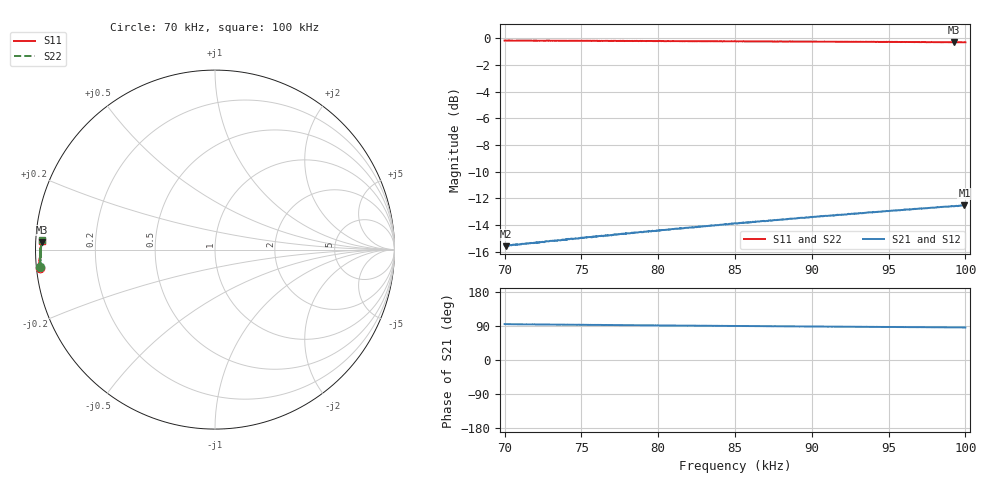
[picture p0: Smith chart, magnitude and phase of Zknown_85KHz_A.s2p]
!Keysight Technologies N9928A: A.12.01
!Date: Monday, January 30, 2023
!Model: N9928A
!Serial: MY58311550
!Caliblation kit: 85033D 3.5mm Calibration Kit
!DUT Connector Gender Port1: male
!DUT Connector Gender Port2: female
!S2P File: Measurements:S11,S21,S12,S22:
# Hz S DB R 50
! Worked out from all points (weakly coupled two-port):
!   1001 points, 70 kHz to 100 kHz, reference 50 ohm
!   highest |S21| = -12.53 dB at 99.94 kHz (marker M1); lowest = -15.6 dB at 70.09 kHz (marker M2)
!   lowest |S11| = -0.3 dB at 99.25 kHz (marker M3), VSWR 56.78, Z = 0.881 + j1.09 ohm
!   |S11| at or under -10 dB: nowhere
!   |S22| runs from -0.3 to -0.2 dB; largest |S21 - S12| = 0.0019
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70000  -0.17 -173.9  -15.53 94.7  -15.62 94.6  -0.20 -174.4
70090  -0.18 -173.9  -15.59 94.6  -15.58 94.2  -0.19 -174.4
71020  -0.17 -174.2  -15.45 94.3  -15.49 94.1  -0.20 -174.7
71350  -0.18 -174.4  -15.39 94.1  -15.44 93.8  -0.20 -174.8
72550  -0.19 -174.8  -15.27 93.7  -15.31 93.8  -0.20 -175.4
73840  -0.18 -175.3  -15.11 93.4  -15.14 93.3  -0.20 -175.7
74170  -0.19 -175.4  -15.06 93.2  -15.09 93.2  -0.21 -175.9
75010  -0.19 -175.6  -14.99 92.8  -15.02 93.0  -0.21 -176.1
76840  -0.20 -176.3  -14.78 92.2  -14.80 92.2  -0.21 -176.8
77620  -0.20 -176.5  -14.69 92.2  -14.70 92.0  -0.21 -176.9
77950  -0.20 -176.7  -14.65 91.8  -14.69 91.9  -0.22 -177.1
78190  -0.20 -176.7  -14.62 91.8  -14.63 91.8  -0.22 -177.1
80020  -0.21 -177.3  -14.43 91.3  -14.41 91.2  -0.22 -177.7
82030  -0.23 -177.9  -14.19 90.7  -14.22 90.7  -0.23 -178.3
85000  -0.22 -178.7  -13.88 89.7  -13.92 89.8  -0.24 -179.2
88240  -0.25 -179.7  -13.59 88.8  -13.58 89.0  -0.26 179.9
90010  -0.25 179.9  -13.43 88.4  -13.43 88.6  -0.26 179.4
95020  -0.27 178.6  -12.96 87.1  -12.98 87.1  -0.29 178.2
96880  -0.28 178.1  -12.78 86.6  -12.81 86.9  -0.30 177.7
99250  -0.31 177.5  -12.61 86.1  -12.61 86.1  -0.31 177.1
99940  -0.30 177.4  -12.53 85.8  -12.55 86.0  -0.31 177.0
100000  -0.30 177.3  -12.53 86.0  -12.55 85.9  -0.31 176.9
